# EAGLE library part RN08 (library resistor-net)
RESISTOR NETWORK
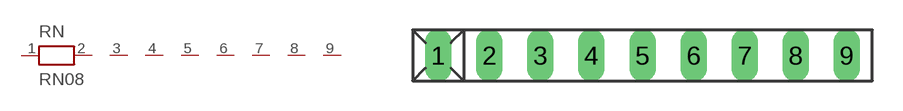
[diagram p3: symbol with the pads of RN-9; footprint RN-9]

Designator prefix RN

## RN08 (OC_FARNELL: unknown; OC_NEWARK: unknown)  [RN-9]
1  1  pas
2  2  pas
3  3  pas
4  4  pas
5  5  pas
6  6  pas
7  7  pas
8  8  pas
9  9  pas

## Footprint RN-9 (pad centres in mm)
RESISTOR NETWORK
drill 0.813 long: 1 -10.16,0; 2 -7.62,0; 3 -5.08,0; 4 -2.54,0; 5 0,0; 6 2.54,0; 7 5.08,0; 8 7.62,0; 9 10.16,0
